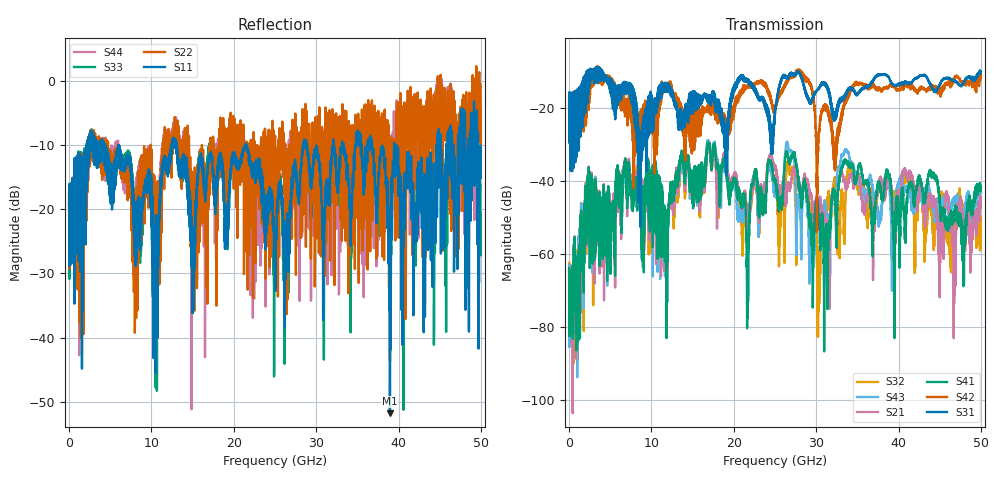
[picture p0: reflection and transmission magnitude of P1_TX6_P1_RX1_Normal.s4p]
!Keysight Technologies,N5225B,MY57041031,A.13.20.10
!Date: Friday, May 31, 2019 11:14:15
!Correction: S11(Full 4 Port(1,2,3,4))
!S12(Full 4 Port(1,2,3,4))
!S13(Full 4 Port(1,2,3,4))
!S14(Full 4 Port(1,2,3,4))
!S21(Full 4 Port(1,2,3,4))
!S22(Full 4 Port(1,2,3,4))
!S23(Full 4 Port(1,2,3,4))
!S24(Full 4 Port(1,2,3,4))
!S31(Full 4 Port(1,2,3,4))
!S32(Full 4 Port(1,2,3,4))
!S33(Full 4 Port(1,2,3,4))
!S34(Full 4 Port(1,2,3,4))
!S41(Full 4 Port(1,2,3,4))
!S42(Full 4 Port(1,2,3,4))
!S43(Full 4 Port(1,2,3,4))
!S44(Full 4 Port(1,2,3,4))
!S4P File: Measurements: <S11,S12,S13,S14>,
!<S21,S22,S23,S24>,
!<S31,S32,S33,S34>,
!<S41,S42,S43,S44>:
# Hz S  dB  R 50.0
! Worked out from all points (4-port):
!   5000 points, 10 MHz to 50 GHz, reference 50 ohm
!   strongest paths, dB at 10 MHz, 12.51 GHz, 25.01 GHz, 37.51 GHz, 50 GHz:
!     S31: -19.4, -15.5, -21.6, -10.8, -9.9
!     S42: -19.5, -14.7, -19.9, -14.9, -10.9
!     S41: -63.8, -43.8, -39.7, -40.7, -41.3
!     S21: -64.6, -44.9, -36.4, -42.8, -44.4
!     S43: -63.0, -44.4, -43.2, -47.4, -41.5
!     S32: -74.1, -45.3, -40.3, -42.0, -50.4
!   lowest |S11| = -51.8 dB at 38.96 GHz (marker M1), VSWR 1.01, Z = 50.2 + j0.159 ohm
!   |S11| at or under -10 dB: 6.02 GHz to 12.47 GHz (6.445 GHz wide, 69.7 % of centre); 13.02 GHz to 21.43 GHz (8.403 GHz wide, 48.8 % of centre); 21.46 GHz to 28.42 GHz (6.959 GHz wide, 27.9 % of centre)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
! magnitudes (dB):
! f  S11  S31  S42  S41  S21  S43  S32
! 10 MHz  -19.4  -19.4  -19.5  -63.8  -64.6  -63.0  -74.1
! 7.07 GHz  -12.3  -13.3  -20.3  -43.3  -44.0  -37.3  -38.8
! 21.68 GHz  -11.1  -12.3  -13.6  -64.8  -51.9  -59.9  -58.2
! 26.66 GHz  -24.2  -11.6  -11.6  -34.6  -40.9  -31.4  -35.4
! 30.3 GHz  -12.3  -14.5  -28.0  -49.3  -46.8  -47.2  -65.1
! 38.96 GHz  -51.8  -12.3  -13.6  -39.4  -39.7  -44.0  -39.9
! 50 GHz  -11.1  -9.9  -10.9  -41.3  -44.4  -41.5  -50.4
